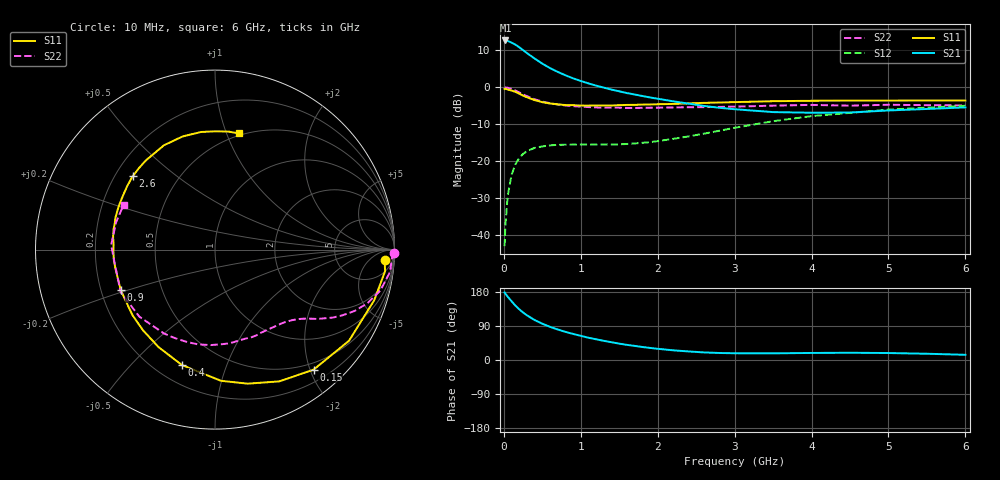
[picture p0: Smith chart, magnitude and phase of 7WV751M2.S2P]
! Infineon Technologies  Discrete & RF Semiconductors
! BFS17W
! Si NPN RF Bipolar Junction Transistor in SOT323
! VCE = 0.75 V  IC = 1.2 mA
! Common Emitter S-Parameters:  August  1999
# GHz  S  MA  R  50
!  f  S11  S21  S12  S22
! GHz  MAG  ANG  MAG  ANG  MAG  ANG  MAG  ANG
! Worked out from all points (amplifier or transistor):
!   36 points, 10 MHz to 6 GHz, reference 50 ohm
!   highest |S21| = 12.6 dB at 20 MHz (marker M1)
!   |S21| within 3 dB of that: start of sweep to 274.6 MHz
!   unconditionally stable (mu >= 1): 881.8 MHz to end of sweep
!   at 250 MHz: K = 0.32, MSG = 14.0 dB, |S12| = -18.0 dB
!   at 1.4 GHz: K = 1.41, MAG = 3.6 dB, |S12| = -15.5 dB
!   at 6 GHz: K = 1.14, MAG = -2.5 dB, |S12| = -5.0 dB
!   S11 on the Smith chart (normalised r, x): 10 MHz: 17, -18; 150 MHz: 0.39, -2.06; 400 MHz: 0.30, -0.71; 900 MHz: 0.28, -0.19; 2.6 GHz: 0.27, +0.36; 6 GHz: 0.48, +1.11
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0.01  0.9462 -3.4  4.271 178.2  0.0071 84.5  0.999 -1.0
0.02  0.9552 -7.2  4.286 175.0  0.0134 84.9  0.9867 -2.8
0.05  0.9311 -17.6  4.226 167.0  0.0339 80.2  0.9836 -7.2
0.1  0.9031 -34.2  4.009 155.2  0.0653 70.3  0.9498 -13.8
0.15  0.8655 -50.6  3.768 143.6  0.0907 60.9  0.9004 -19.4
0.2  0.8169 -64.0  3.472 133.9  0.1106 54.0  0.85 -23.7
0.25  0.7688 -76.3  3.176 125.3  0.1254 47.6  0.7986 -27.3
0.3  0.7317 -87.4  2.894 118.0  0.1367 43.2  0.7576 -30.0
0.4  0.6693 -105.9  2.441 105.4  0.1515 36.1  0.6874 -34.2
0.5  0.6276 -120.1  2.084 95.8  0.1582 31.4  0.6398 -36.9
0.6  0.6024 -131.8  1.813 87.5  0.1637 28.3  0.6078 -39.5
0.7  0.5872 -141.6  1.612 80.5  0.1662 26.4  0.5842 -42.2
0.9  0.5715 -157.0  1.319 68.8  0.1674 24.6  0.5542 -47.8
1.1  0.5645 -169.1  1.126 58.7  0.1678 24.8  0.5389 -53.9
1.6  0.5762 168.9  0.833 40.0  0.1709 31.3  0.5244 -70.9
2.2  0.5943 149.7  0.645 25.6  0.2003 42.4  0.5325 -92.6
2.6  0.6145 138.4  0.559 20.0  0.2354 46.9  0.538 -107.3
3.5  0.6471 116.1  0.461 17.6  0.3472 46.1  0.5632 -138.4
4  0.6557 106.0  0.452 18.6  0.4065 41.1  0.5766 -155.7
4.5  0.6599 96.8  0.455 19.1  0.45 35.5  0.5634 -170.7
5.5  0.6617 83.5  0.508 16.5  0.53 25.0  0.5719 164.6
6  0.6607 78.4  0.534 13.7  0.562 19.9  0.5672 153.8
